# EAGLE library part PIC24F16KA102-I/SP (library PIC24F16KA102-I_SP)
Flash Microcontrollers
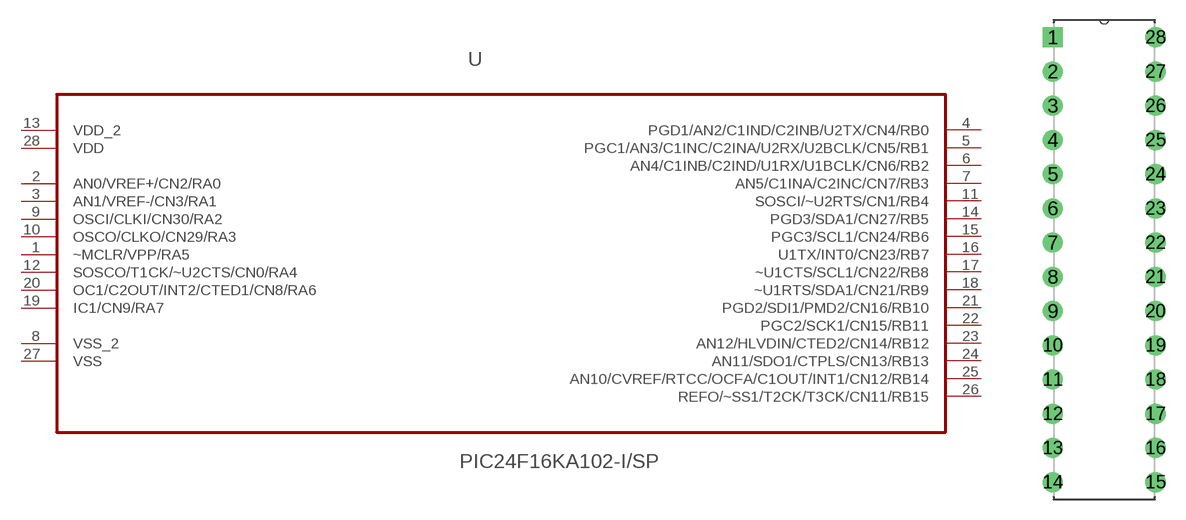
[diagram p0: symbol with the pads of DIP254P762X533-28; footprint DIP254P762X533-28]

Designator prefix -

## PIC24F16KA102-I/SP (AVAILABILITY: Bad; DESCRIPTION: 28-Pin, 16KB Flash, 2KB RAM, 512B EEPROM, 16 MIPS, 19 I/O, 16-Bit PIC24F Family; MF: Microchip; MP: PIC24F16KA102-I/SP; PACKAGE: SPDIP-28 Microchip; PRICE: 2.38 USD)  [DIP254P762X533-28]
1  ~MCLR/VPP/RA5
2  AN0/VREF+/CN2/RA0
3  AN1/VREF-/CN3/RA1
4  PGD1/AN2/C1IND/C2INB/U2TX/CN4/RB0
5  PGC1/AN3/C1INC/C2INA/U2RX/U2BCLK/CN5/RB1
6  AN4/C1INB/C2IND/U1RX/U1BCLK/CN6/RB2
7  AN5/C1INA/C2INC/CN7/RB3
8  VSS_2  pas
9  OSCI/CLKI/CN30/RA2
10  OSCO/CLKO/CN29/RA3
11  SOSCI/~U2RTS/CN1/RB4
12  SOSCO/T1CK/~U2CTS/CN0/RA4
13  VDD_2  pas
14  PGD3/SDA1/CN27/RB5
15  PGC3/SCL1/CN24/RB6
16  U1TX/INT0/CN23/RB7
17  ~U1CTS/SCL1/CN22/RB8
18  ~U1RTS/SDA1/CN21/RB9
19  IC1/CN9/RA7
20  OC1/C2OUT/INT2/CTED1/CN8/RA6
21  PGD2/SDI1/PMD2/CN16/RB10
22  PGC2/SCK1/CN15/RB11
23  AN12/HLVDIN/CTED2/CN14/RB12
24  AN11/SDO1/CTPLS/CN13/RB13
25  AN10/CVREF/RTCC/OCFA/C1OUT/INT1/CN12/RB14
26  REFO/~SS1/T2CK/T3CK/CN11/RB15
27  VSS  pas
28  VDD  pwr

## Footprint DIP254P762X533-28 (pad centres in mm)
drill 0.991 square: 1 -7.62,33.02
drill 0.991: 2 -7.62,30.48; 3 -7.62,27.94; 4 -7.62,25.4; 5 -7.62,22.86; 6 -7.62,20.32; 7 -7.62,17.78; 8 -7.62,15.24; 9 -7.62,12.7; 10 -7.62,10.16; 11 -7.62,7.62; 12 -7.62,5.08; 13 -7.62,2.54; 14 -7.62,0; 15 0,0; 16 0,2.54; 17 0,5.08; 18 0,7.62; 19 0,10.16; 20 0,12.7; 21 0,15.24; 22 0,17.78; 23 0,20.32; 24 0,22.86; 25 0,25.4; 26 0,27.94; 27 0,30.48; 28 0,33.02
